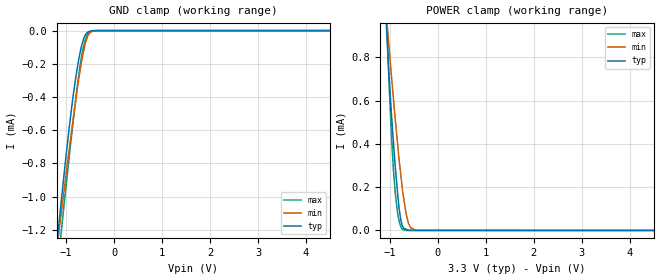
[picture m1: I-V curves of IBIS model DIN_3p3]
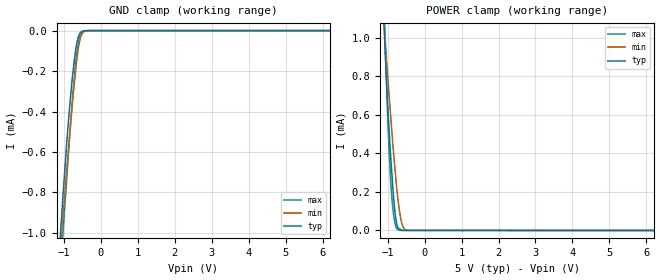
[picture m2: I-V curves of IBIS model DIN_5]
|Texas Instruments Incorporated
|14-Bit, Dual-Channel, Ultralow-glitch, Low-power, Voltage-output DAC
|   With 2/5-V, 2PPM/C Internal Reference in a Tiny 3 mm x 3 mm QFN
| Marketing part#   Digital Voltage Range   Package-type   #pins
|DAC8162SDGS   2.7 to 5.5   MSOP   10
|DAC8162SDSC   2.7 to 5.5   QFN   10
[IBIS Ver]   4.0
[File name]   dac8162.ibs
[File Rev]   2.0
[Date]   02/28/2011
[Source]   Texas Instruments Incorporated.
   Analog-eLab, HPA
   12500 TI Blvd
   Dallas, TX -75243
   For Support e-mail: elab_ibis@list.ti.com
[Notes]   Revision History:
   1.0: 08/17/2010
   - Initial version of the model
   - Initial Model generated from simulations in TISPICED
   - Model names with a trailing _18 contains the model for
   1.8V (1.625V and 1.96V).
   - Model names with a trailing _3 contains the model for
   3V (2.7V and 3.3V).
   - Model names with trailing _5 contains
   the model for 5V (4.75V and 5.25V) operation.
   - Model not matched to measurements
   - Ignore warnings related to min and max values of ccomp,
   The device process of these products is CMOS. The ccomp
   values are based on PVT variations as seen in simulations
   - C_comp: Ignore warnings related to typical values not being
   in between the minimum and maximum values for SDA_3
   SDA_5. The c_comp values are
   a mathematical average between the buffer's ON state and
   OFF state.
   2.0: 02/24/2011
   - Added c_comp values in corrrect typ, min, and max order.
   - Modified buffer names to reflect silicon labeling
   - 1.8V option removed due to silicon limits
   - Replaced NC buffer with TERM buffer to reflect analog pins
   - Model names with a trailing _3p3 contains the model for
   3.3V (3V and 3.6V).
   - Model names with trailing _5 contains
   the model for 5V (4.5V and 5.5V) operation.
   2.1: 02/28/2011
   - updated Vinl and Vinh per designer's feedback
[Disclaimer]
 This product is designed as an aid for customers of Texas Instruments.
 No warranties, either expressed or implied, with respect to this third
 party software (if any) or with respect to its fitness for any
 particular purpose is claimed by Texas Instruments or the author. The
 software (if any) is provided solely on an "as is" basis. The entire
 risk as to its quality and performance is with the customer
[Copyright] (C) Copyright 2010 Texas Instruments Incorporated.
   All rights reserved.
|   DAC8162
[Component]   dac8162sdsr  |QFN package - 10
[Manufacturer] TI
[Package]
| variable   typ   min   max
R_pkg  0.048703   0.044430   0.062040
L_pkg  0.729825nH 0.667840nH 0.945020nH
C_pkg  0.133535pF 0.120760pF 0.154700pF
[Pin] signal_name  model_name  R_pin  L_pin C_pin
1   VOUTA   TERM   0.04443  0.66784nH  0.12076pF
2   VOUTB   TERM   0.06204  0.94502nH  0.15470pF
3   GND   GND   0.05294  0.79766nH  0.14696pF
4   _LDAC   DIN   0.04736  0.71008nH  0.14053pF
5   _CLR   DIN   0.04486  0.67449nH  0.12270pF
6   _SYNC   DIN   0.04503  0.66912nH  0.12224pF
7   SCLK   DIN   0.04601  0.68159nH  0.13883pF
8   DIN   DIN   0.05308  0.79370nH  0.14526pF
9   AVDD   POWER   0.04562  0.67535nH  0.13655pF
10  VREFIN_VREFOUT  TERM   0.04681  0.69676nH  0.12326pF
[Component]   dac8162sdgs  |MSOP package - 10
[Manufacturer] TI
[Package]
| variable   typ   min   max
R_pkg  0.053909   0.050510   0.065160
L_pkg  1.250835nH 1.192710nH 1.442660nH
C_pkg  0.277796pF 0.258920pF 0.305020pF
[Pin] signal_name  model_name  R_pin  L_pin C_pin
1   VOUTA   TERM   0.05066  1.20497nH  0.25892pF
2   VOUTB   TERM   0.06516  1.44266nH  0.30502pF
3   GND   GND   0.05727  1.30607nH  0.29591pF
4   _LDAC   DIN   0.05243  1.22369nH  0.29066pF
5   _CLR   DIN   0.05051  1.20299nH  0.26048pF
6   _SYNC   DIN   0.05067  1.19724nH  0.26062pF
7   SCLK   DIN   0.05131  1.19271nH  0.29175pF
8   DIN   DIN   0.05744  1.30248nH  0.29417pF
9   AVDD   POWER   0.05139  1.19797nH  0.28622pF
10  VREFIN_VREFOUT  TERM   0.05309  1.23994nH  0.26075pF
|   Model Selectors
[Model Selector]  DIN
DIN_3p3  3.3V digital input
DIN_5   5V digital input
|NOTES   Model DIN split into two Models DIN_3p3 and DIN_5
|   to accomodate vast voltage range of 2.7V - 5.5V
|   DIN_3p3 operates in voltage range of 3.0 - 3.3 - 3.6
|   DIN_5 operates in voltage range of 4.5 - 5.0 - 5.5
|   The pin frequency for Model DIN is 50MHz
|   This is referenced with datasheet
[Model Selector]  TERM
TERM_3p3  3.3V terminator
TERM_5   5V terminator
|   DIN_3p3  3.3V digital input Model
[Model]   TERM_3p3
Model_type   Terminator
C_comp   1e-20   1e-20   1e-20
[Voltage Range]   3.3   3   3.6
[Temperature Range]   27   125   -40
[GND Clamp Reference]   0   0   0
|   DIN_5  5V digital input Model
[Model]   TERM_5
Model_type   Terminator
C_comp   1e-20   1e-20   1e-20
[Voltage Range]   5   4.5   5.5
[Temperature Range]   27   125   -40
[GND Clamp Reference]   0   0   0
| Models and submodels in the file (4): DIN_3p3 (Input), DIN_5 (Input), TERM_3p3 (Terminator), TERM_5 (Terminator)
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|NOTES   Model TERM split into two Models TERM_3p3 and TERM_5
|   to accomodate vast voltage range of 2.7V - 5.5V
|   TERM_3p3 operates in voltage range of 3.0 - 3.3 - 3.6
|   TERM_5 operates in voltage range of 4.5 - 5.0 - 5.5
|   DIN_3p3  3.3V digital input Model
[Model]   DIN_3p3
Model_type   Input
Vinl = 0.8
Vinh = 2.2
|   typ   min   max
|   (nom PVT)   (Fast PVT)   (slow PVT)
C_comp   2.61868E-13   2.43265E-13   3.59268E-13
|C_comp from L-C Tank method (L=1nH)
|Resonant Frequency(Hz)   9.84E+09   10.2E+09   8.40E+09
|C_comp   4.3970090e-13  4.0118260e-13  4.7940920e-13
|C_comp from frequency method, 50 MHz
| Where nom  PVT is Nominal Process,  3.3V,  27C
|   Fast PVT is Strong Process,   3.6V,  -40C
|   Slow PVT is Weak Process,   3.0V,  125C
[Voltage Range]   3.3   3   3.6
[Temperature Range]   27   125   -40
[Power Clamp Reference]   3.3   3   3.6
[GND Clamp Reference]   0   0   0
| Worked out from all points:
|   GND clamp passes 1 mA (typ) near -1.09 V on its own axis
|   POWER clamp passes 1 mA (typ) near -1.08 V on its own axis
[GND Clamp]
|   Voltage   I(typ)   I(min)   I(max)
-3.3V     -7.772mA   -6.534mA   -9.257mA
-1.173V   -1.23mA    -1.267mA   -1.412mA
-1.141V   -1.14mA    -1.19mA    -1.323mA
-1.12V    -1.08mA    -1.14mA    -1.264mA
-1.086V   -984.2uA   -1.062mA   -1.169mA
-932.5mV  -576.9uA   -707.4uA   -751.8uA
-801mV    -286.3uA   -421.5uA   -416.7uA
-665.6mV  -80.14uA   -167.8uA   -135.4uA
-605mV    -29.95uA   -84.25uA   -59.96uA
-541mV    -7.514uA   -28.19uA   -17.48uA
-345.6mV  -254.7nA   -205.3nA   -262.5nA
6.6V      0A         0A         0A
[POWER Clamp]
|   Voltage   I(typ)   I(min)   I(max)
-3.3V     13.6mA     10.98mA    16.4mA
-1.062V   904.8uA    974.4uA    939.1uA
-1.039V   807.3uA    907uA      810.7uA
-965.1mV  530.5uA    710.4uA    431.6uA
-922.7mV  399uA      600.1uA    270.4uA
-888.4mV  296.6uA    515.9uA    174.6uA
-838mV    168.6uA    396.8uA    80.73uA
-782.5mV  63.4uA     276.8uA    24.14uA
-734.7mV  19.53uA    183uA      4.619uA
-612.2mV  1.251uA    33.54uA    430.2nA
-443.6mV  265.7nA    419.5nA    420.2nA
6.6V      0A         0A         0A
|   DIN_5   5V digital input
[Model]   DIN_5
Model_type   Input
Vinl = 0.8
Vinh = 3.1
|   typ   min   max
|   (nom PVT)   (Fast PVT)   (slow PVT)
C_comp   2.50082E-13   2.31249E-13   2.51233E-13
|C_comp from L-C Tank method (L=1nH)
|Resonant Frequency(Hz)   10.0693E+09   10.4713E+09   10.046E+09
|C_comp   4.2241620e-13  3.8549500e-13  4.6040220e-13
|C_comp from frequency method, 50 MHz
| Where nom  PVT is Nominal Process,  5V,  27C
|   Fast PVT is Strong Process,   5.5V,  -40C
|   Slow PVT is Weak Process,   4.5V,  125C
[Voltage Range]   5   4.5   5.5
[Temperature Range]   27   125   -40
[Power Clamp Reference]   5   4.5   5.5
[GND Clamp Reference]   0   0   0
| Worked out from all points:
|   GND clamp passes 1 mA (typ) near -1.09 V on its own axis
|   POWER clamp passes 1 mA (typ) near -1.08 V on its own axis
[GND Clamp]
|   Voltage   I(typ)   I(min)   I(max)
-5V       -13.1mA    -10.82mA   -15.79mA
-1.118V   -1.072mA   -1.136mA   -1.257mA
-1.053V   -892.6uA   -982.7uA   -1.074mA
-1.027V   -822.6uA   -924.1uA   -1.006mA
-853.8mV  -394.2uA   -533.9uA   -547.3uA
-782.2mV  -250.9uA   -382.4uA   -372.9uA
-711mV    -134.3uA   -246.2uA   -216.6uA
-671.7mV  -84.44uA   -176.4uA   -145uA
-608.1mV  -30.87uA   -86.63uA   -63.06uA
-549.6mV  -9.224uA   -33.4uA    -21.71uA
-493.8mV  -2.32uA    -12.19uA   -5.19uA
10V       0A         0A         0A
[POWER Clamp]
|   Voltage   I(typ)   I(min)   I(max)
-5V       23.59mA    19.04mA    28.46mA
-1.103V   1.088mA    1.091mA    1.184mA
-1.072V   942.8uA    1.003mA    994.2uA
-991.5mV  622.8uA    777.5uA    554.4uA
-956.8mV  506uA      689.8uA    396.4uA
-906.2mV  350.4uA    562.1uA    220.4uA
-866.3mV  239.7uA    461.5uA    127.7uA
-819.7mV  127.8uA    356.5uA    57.68uA
-735.9mV  20.35uA    185uA      4.811uA
-621.9mV  2.687uA    40.47uA    350.2nA
-434.5mV  236nA      320.5nA    344nA
10V       0A         0A         0A
